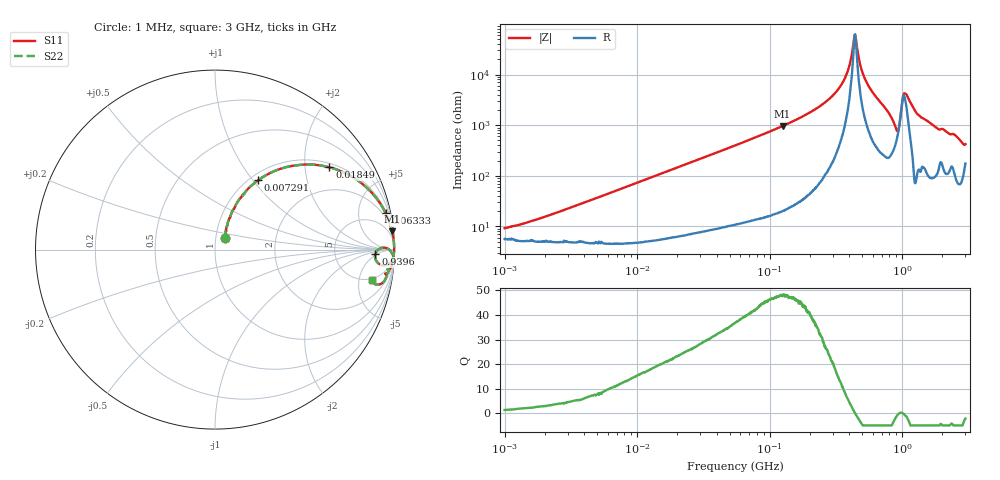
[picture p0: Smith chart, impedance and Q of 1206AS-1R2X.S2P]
!s-Parameter Generated by FASTRON Sdn. Bhd.
!FASTRON P/N : 1206AS-1R2X
!Keysight Technologies: E4991B_MY54100416_A.01.15
!Date created: Thu Nov 16 13:44:16 2023
!Version  : Rev00 Thu Nov 16 13:44:16 2023
!Data & Calibration Information:
!Freq	S11	S21	S12	S22
!PortZ  Port1:50+j0  Port2:50+j0
!When reading reference impedance value at option line is always used.
! Remarks : This data is being provided solely for informational purposes.
# Hz S dB R 50
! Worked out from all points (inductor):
!   1601 points, 1 MHz to 3 GHz, reference 50 ohm
!   read as one part in series: L = 1.17 uH near 2.097 MHz
!   highest Q = 47.9 at 125.1 MHz (marker M1), where L = 1.22 uH
!   self-resonance near 439.1 MHz
!   S11 on the Smith chart (normalised r, x): 1 MHz: 1.11, +0.15; 7.291 MHz: 1.09, +1.07; 18.49 MHz: 1.12, +2.69; 63.33 MHz: 1.24, +9.21; 939.6 MHz: 17, -4; 3 GHz: 4.51, -7.67
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1000000  -21.17 48.4  -0.50 -4.0  -0.50 -4.0  -21.17 48.4
3804036  -11.69 65.0  -0.72 -14.9  -0.72 -14.9  -11.69 65.0
7290557  -6.83 58.1  -1.39 -27.0  -1.39 -27.0  -6.83 58.1
1.447069e7  -3.00 42.1  -3.46 -45.0  -3.46 -45.0  -3.00 42.1
1.849167e7  -2.10 35.7  -4.66 -51.7  -4.66 -51.7  -2.10 35.7
5.477226e7  -0.32 14.0  -12.30 -74.4  -12.30 -74.4  -0.32 14.0
6.33262e7  -0.25 12.2  -13.52 -76.4  -13.52 -76.4  -0.25 12.2
1.250659e8  -0.07 5.9  -19.72 -82.9  -19.72 -82.9  -0.07 5.9
2.083556e8  -0.02 3.0  -25.52 -85.5  -25.52 -85.5  -0.02 3.0
3.48855e8  -0.01 0.9  -36.14 -84.1  -36.14 -84.1  -0.01 0.9
3.91407e8  -0.01 0.5  -41.91 -79.1  -41.91 -79.1  -0.01 0.5
4.282981e8  -0.01 0.1  -52.27 -50.3  -52.27 -50.3  -0.01 0.1
4.413523e8  -0.01 -0.0  -55.86 3.2  -55.86 3.2  -0.01 -0.0
4.902556e8  -0.02 -0.4  -42.49 75.6  -42.49 75.6  -0.02 -0.4
5.311214e8  -0.02 -0.7  -37.62 80.5  -37.62 80.5  -0.02 -0.7
7.925923e8  -0.08 -3.2  -24.90 79.2  -24.90 79.2  -0.08 -3.2
8.982141e8  -0.55 -5.3  -19.28 53.1  -19.28 53.1  -0.55 -5.3
9.395906e8  -0.97 -1.5  -19.24 12.8  -19.24 12.8  -0.97 -1.5
1.01283e9  -0.24 -0.1  -31.25 4.1  -31.25 4.1  -0.24 -0.1
1.059487e9  -0.15 -0.9  -32.58 43.5  -32.58 43.5  -0.15 -0.9
1.353887e9  -0.06 -3.7  -23.78 81.5  -23.78 81.5  -0.06 -3.7
3e9  -0.98 -11.1  -13.48 54.3  -13.48 54.3  -0.98 -11.1
